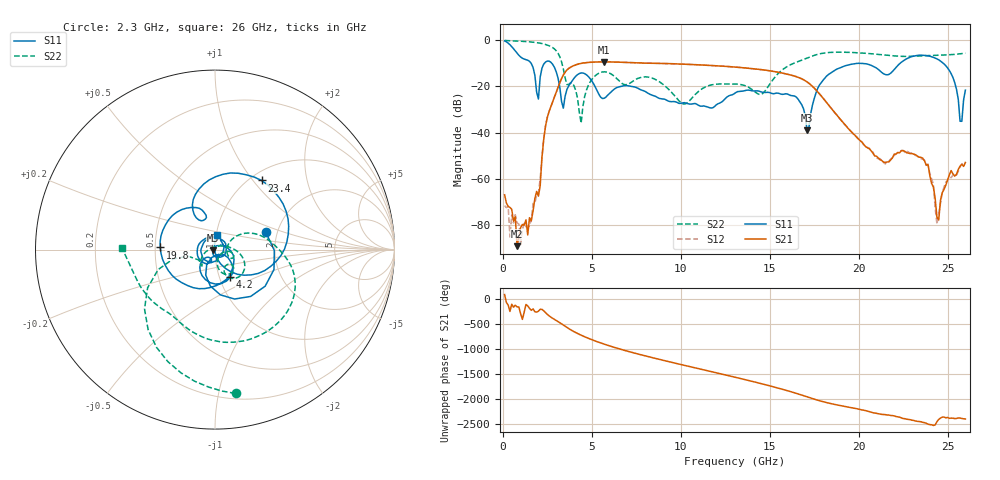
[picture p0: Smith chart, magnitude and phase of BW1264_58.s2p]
!Keysight Technologies,N5245B,MY57181159,A.13.60.06
!Date: Friday, December 18, 2020 23:55:06
!Correction: S11(Full 2 Port(1,2))
!S21(Full 2 Port(1,2))
!S12(Full 2 Port(1,2))
!S22(Full 2 Port(1,2))
!S2P File: Measurements: S11, S21, S12, S22:
# Hz S  dB  R 50
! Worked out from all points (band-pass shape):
!   260 points, 100 MHz to 26 GHz, reference 50 ohm
!   highest |S21| = -9.53 dB at 5.7 GHz (marker M1); lowest = -89.0 dB at 800 MHz (marker M2)
!   |S21| within 3 dB of the highest: 3.679 GHz to 14.12 GHz (10.44 GHz wide, 117 % of centre)
!   lowest |S11| = -39.0 dB at 17.1 GHz (marker M3), VSWR 1.02, Z = 48.9 - j0.334 ohm
!   |S11| at or under -10 dB: 1.574 GHz to 2.355 GHz (780.9 MHz wide, 39.7 % of centre); 2.736 GHz to 22.35 GHz (19.62 GHz wide, 156 % of centre); 24.73 GHz to end of sweep
!   |S22| runs from -36.0 to -0.3 dB; largest |S21 - S12| = 0.00072
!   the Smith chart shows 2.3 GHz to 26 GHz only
!   S11 on the Smith chart (normalised r, x): 2.3 GHz: 1.74, +0.37; 4.2 GHz: 1.13, -0.36; 19.8 GHz: 0.53, +0.01; 23.4 GHz: 1.13, +1.10; 26 GHz: 1.01, +0.16
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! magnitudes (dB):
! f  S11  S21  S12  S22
! 100 MHz  -0.5  -66.8  -71.5  -0.3
! 800 MHz  -5.8  -89.0  -79.0  -0.6
! 1.5 GHz  -9.3  -76.7  -80.1  -0.9
! 2 GHz  -25.5  -67.4  -66.1  -1.4
! 2.3 GHz  -10.5  -42.8  -42.6  -1.8
! 3.4 GHz  -29.5  -15.2  -15.2  -12.5
! 4.2 GHz  -15.0  -10.6  -10.6  -25.3
! 4.5 GHz  -14.3  -10.1  -10.0  -28.9
! 5.7 GHz  -25.2  -9.5  -9.5  -13.8
! 8.8 GHz  -25.3  -10.2  -10.2  -18.1
! 13.1 GHz  -22.7  -11.8  -11.8  -19.1
! 16.4 GHz  -24.3  -15.7  -15.7  -10.0
! 17.1 GHz  -39.0  -18.2  -18.2  -7.9
! 17.4 GHz  -28.3  -20.1  -20.1  -7.0
! 19.8 GHz  -10.3  -41.2  -41.4  -5.5
! 21.7 GHz  -15.0  -52.7  -52.5  -6.8
! 23.4 GHz  -6.7  -50.6  -51.0  -7.0
! 24.2 GHz  -7.6  -63.4  -62.3  -6.8
! 24.4 GHz  -8.2  -76.5  -79.4  -6.7
! 25.3 GHz  -16.3  -57.8  -58.3  -6.4
! 25.7 GHz  -35.1  -54.5  -54.7  -6.1
! 26 GHz  -21.7  -52.9  -52.7  -5.7
